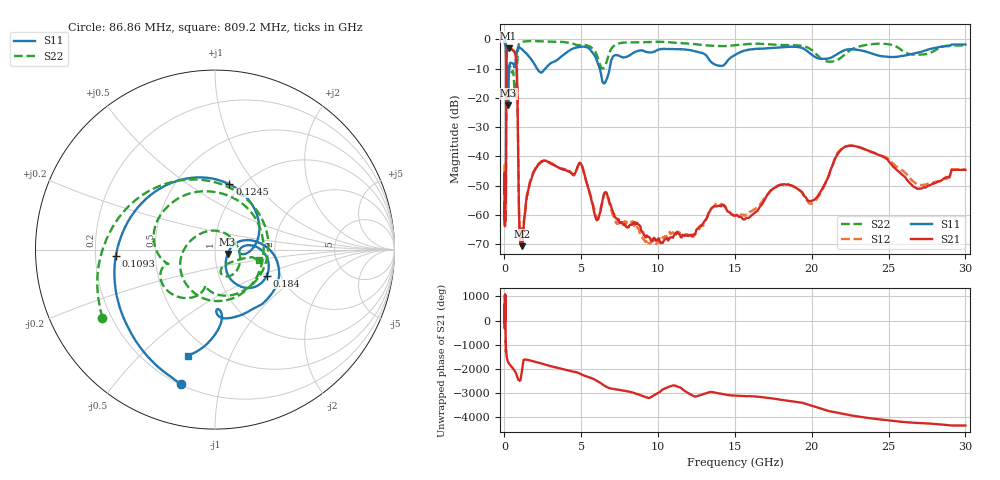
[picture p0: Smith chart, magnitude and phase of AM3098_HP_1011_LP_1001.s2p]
! Date/Time: Thu, Feb 28, 2019 8:43 AM
! Network Analyzer: Agilent Technologies E8364B Rev: A.07.50.67
! Sweep from 0.010 to 30.000 GHz, 1601 Points, Sweep Type: LOG
! Power Supply: 5.022 V, 0.002 A
# Hz S DB R 50
!freq MagS11 AngS11 MagS21 AngS21 MagS12 AngS12 MagS22 AngS22
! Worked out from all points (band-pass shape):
!   1601 points, 10 MHz to 30 GHz, reference 50 ohm
!   highest |S21| = -3.09 dB at 265.1 MHz (marker M1); lowest = -70.8 dB at 1.132 GHz (marker M2)
!   |S21| within 3 dB of the highest: 137.5 MHz to 736.4 MHz (598.9 MHz wide, 137 % of centre)
!   lowest |S11| = -22.6 dB at 242.3 MHz (marker M3), VSWR 1.16, Z = 57.5 - j2.83 ohm
!   |S11| at or under -10 dB: 191.2 MHz to 306.3 MHz (115.1 MHz wide, 46.3 % of centre); 2.117 GHz to 2.667 GHz (549.5 MHz wide, 23 % of centre); 6.201 GHz to 6.845 GHz (643.5 MHz wide, 9.86 % of centre)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
!   |S22| runs from -19.8 to -0.5 dB; largest |S21 - S12| = 0.0097
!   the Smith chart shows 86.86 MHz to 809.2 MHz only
!   S11 on the Smith chart (normalised r, x): 86.86 MHz: 0.20, -0.76; 109.3 MHz: 0.29, -0.03; 124.5 MHz: 0.88, +0.74; 184 MHz: 1.70, -0.55; 809.2 MHz: 0.38, -0.71
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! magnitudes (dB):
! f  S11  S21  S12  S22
! 10 MHz  -0.3  -46.1  -42.7  -0.6
! 38.04 MHz  -0.4  -60.9  -60.5  -0.9
! 86.86 MHz  -2.2  -54.3  -54.8  -2.7
! 96 MHz  -3.3  -51.9  -57.5  -3.7
! 109.3 MHz  -5.1  -33.9  -33.8  -6.4
! 124.5 MHz  -8.6  -12.9  -12.9  -10.6
! 144.7 MHz  -17.2  -5.0  -5.0  -13.7
! 184 MHz  -9.8  -3.8  -3.7  -9.1
! 242.3 MHz  -22.6  -3.1  -3.1  -11.3
! 265.1 MHz  -16.0  -3.1  -3.0  -10.8
! 550.5 MHz  -8.2  -3.8  -3.8  -10.8
! 809.2 MHz  -4.3  -11.8  -11.8  -11.9
! 973.8 MHz  -2.7  -64.5  -64.8  -1.3
! 1.132 GHz  -3.3  -70.8  -65.7  -0.8
! 2.084 GHz  -9.7  -43.8  -43.6  -0.6
! 4.927 GHz  -2.5  -42.2  -42.2  -1.9
! 6.521 GHz  -14.9  -52.6  -52.5  -9.4
! 7.926 GHz  -6.0  -64.2  -63.0  -1.0
! 12.13 GHz  -3.7  -67.0  -66.2  -1.4
! 20.1 GHz  -5.6  -55.1  -55.8  -4.0
! 22.67 GHz  -3.4  -36.4  -36.4  -3.2
! 30 GHz  -1.7  -44.6  -44.4  -2.0
